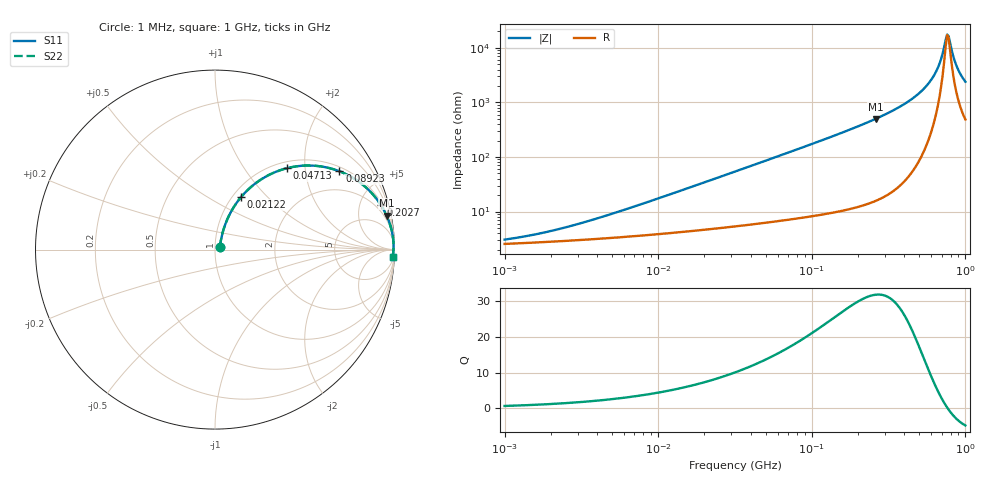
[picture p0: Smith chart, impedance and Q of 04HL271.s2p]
! Coilcraft 0402HL-271 Chip Inductor
! 20 July 2012
# MHz S MA R 50
!Freq  MagS11  AngS11  MagS21  AngS21  MagS12  AngS12  MagS22  AngS22
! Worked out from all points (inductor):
!   304 points, 1 MHz to 1 GHz, reference 50 ohm
!   read as one part in series: L = 270 nH near 6.196 MHz
!   highest Q = 31.9 at 260.5 MHz (marker M1), where L = 305 nH
!   self-resonance near 760.7 MHz
!   S11 on the Smith chart (normalised r, x): 1 MHz: 1.05, +0.03; 21.22 MHz: 1.09, +0.72; 47.13 MHz: 1.12, +1.61; 89.23 MHz: 1.16, +3.07; 202.7 MHz: 1.25, +7.40; 1 GHz: 11, -47
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1  0.02986 32.7  0.975 -0.9  0.975 -0.9  0.02986 32.7
1.768173  0.03958 45.8  0.9728 -1.7  0.9728 -1.7  0.03958 45.8
3.19853  0.06021 57.9  0.9693 -3.0  0.9693 -3.0  0.06021 57.9
10  0.1653 67.9  0.9503 -9.3  0.9503 -9.3  0.1653 67.9
21.21938  0.3281 63.6  0.903 -19.0  0.903 -19.0  0.3281 63.6
31.9853  0.4607 57.1  0.8435 -27.3  0.8435 -27.3  0.4607 57.1
47.12673  0.605 48.5  0.7517 -37.1  0.7517 -37.1  0.605 48.5
89.22674  0.8193 32.2  0.5333 -54.9  0.5333 -54.9  0.8193 32.2
102.306  0.8536 28.8  0.4825 -58.5  0.4825 -58.5  0.8536 28.8
202.7359  0.9574 15.0  0.2587 -73.1  0.2587 -73.1  0.9574 15.0
260.5203  0.9747 11.2  0.195 -77.0  0.195 -77.0  0.9747 11.2
319.853  0.9839 8.6  0.1497 -79.5  0.1497 -79.5  0.9839 8.6
460.645  0.9928 4.7  0.08118 -82.6  0.08118 -82.6  0.9928 4.7
591.9394  0.995 2.3  0.04019 -81.7  0.04019 -81.7  0.995 2.3
633.8408  0.9951 1.7  0.02961 -79.7  0.02961 -79.7  0.9951 1.7
678.7083  0.995 1.1  0.0193 -74.6  0.0193 -74.6  0.995 1.1
710.3709  0.9949 0.7  0.01275 -66.0  0.01275 -66.0  0.9949 0.7
760.6557  0.9945 0.1  0.005653 -13.0  0.005653 -13.0  0.9945 0.1
778.1962  0.9943 -0.1  0.006092 21.0  0.006092 21.0  0.9943 -0.1
833.2822  0.9936 -0.7  0.01408 62.8  0.01408 62.8  0.9936 -0.7
872.1558  0.9931 -1.1  0.02068 69.9  0.02068 69.9  0.9931 -1.1
1000  0.9907 -2.3  0.04145 75.9  0.04145 75.9  0.9907 -2.3
